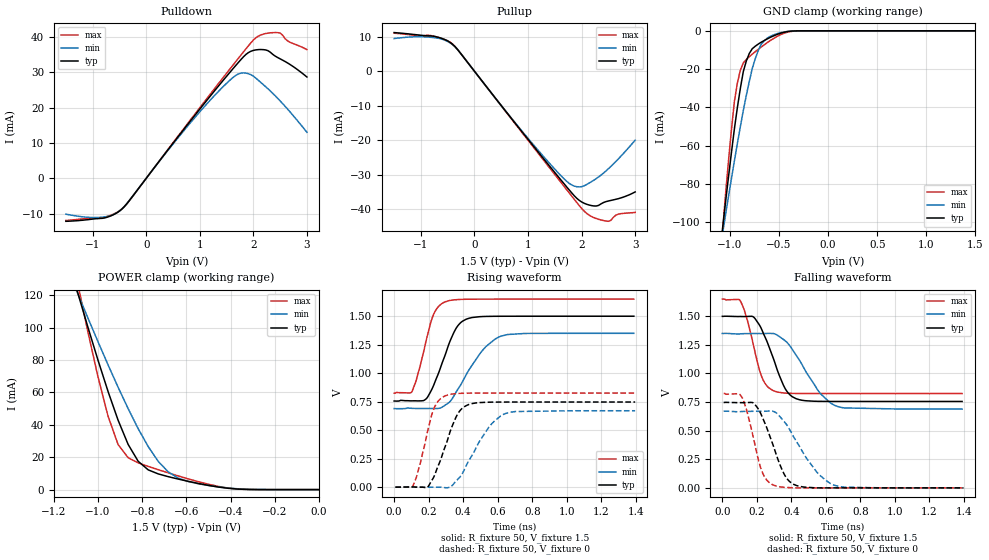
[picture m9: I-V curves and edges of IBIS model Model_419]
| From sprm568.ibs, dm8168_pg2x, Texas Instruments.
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| Model based on original model for BSHTLTCSCDDVGPBFZ
|   Sub model SLOW_8MA_10PER_N_1P5
[model]   Model_419
|[Description]  [1.5V-3-STATE-X-SLOW:8MA, IND, 10%]
|   Slow slew rate (SR[1:0] = "01"), 1.00 * RExt = 1.000 * Iout
|   (I[2:0] = "011"), 8mA nominal with Rext = 50R, ,Industrial
|   temperature range (-40C to 125C, 25C nominal),10% power supply
|   tolerance
|[Input Load]
|[Output Drive] SLOW:8MA
|Voltage   1.5V
|Mode   3-STATE
Model_type   3-state
Polarity   Non-Inverting
Enable   Active-Low
Cref =  15.0000pF
Rref =  100.0000M
Vref =  0V
Vmeas =  0.75
C_comp   1.5249p   1.4275p   1.6205p
[Model Spec]
[Temperature Range]   25   125   -40
[Voltage Range]   1.5   1.35   1.65
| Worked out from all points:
|   slope of the pulldown table from 0 to 0.225 V, typ, clamps not added: 50.1 ohm
|   slope of the pullup table from 0 to 0.225 V, typ, clamps not added: 50.1 ohm
|   GND clamp passes 1 mA (typ) near -0.47 V on its own axis
|   POWER clamp passes 1 mA (typ) near -0.42 V on its own axis
|   rising waveform, R_fixture 50, V_fixture 1.5: 20-80 % time 112ps typ, 168ps min, 83.6ps max; typ from 0.756 V to 1.5 V
|   rising waveform, R_fixture 50, V_fixture 0: 20-80 % time 108ps typ, 154ps min, 80.5ps max; typ from 0 V to 0.747 V
|   falling waveform, R_fixture 50, V_fixture 1.5: 20-80 % time 114ps typ, 168ps min, 82.8ps max; typ from 1.5 V to 0.755 V
|   falling waveform, R_fixture 50, V_fixture 0: 20-80 % time 111ps typ, 170ps min, 80.4ps max; typ from 0.746 V to 0 V
[POWER_clamp]
-1.5V     321.6mA    260.6mA    415.8mA
-1.091V   121.1mA    120.8mA    126.6mA
-1.076V   114.1mA    115.8mA    116.8mA
-1V       79.88mA    91.3mA     69.56mA
-954.5mV  60.58mA    77.05mA    45.34mA
-909.1mV  42.84mA    63.2mA     27.8mA
-818.2mV  17.47mA    37.6mA     16.51mA
-772.7mV  12.19mA    26.53mA    14.33mA
-681.8mV  7.985mA    10.89mA    10.33mA
-590.9mV  5.092mA    4.952mA    6.596mA
-363.6mV  298.9uA    465.6uA    298.1uA
0V        1.518nA    23.05nA    396.5pA
[Pulldown]
-1.5V     -12.15mA   -10.14mA   -11.93mA
-772.7mV  -11.18mA   -10.9mA    -10.98mA
-590.9mV  -10.12mA   -10.11mA   -9.968mA
-409.1mV  -8.017mA   -7.951mA   -8.019mA
954.5mV   18.69mA    17.99mA    19.06mA
1.455V    28.01mA    26.18mA    28.82mA
1.727V    32.86mA    29.54mA    34.05mA
2V        36.15mA    28.87mA    39.08mA
2.318V    35.62mA    24.67mA    41.12mA
2.5V      33.77mA    21.88mA    41.05mA
2.636V    32.63mA    19.61mA    38.86mA
3V        28.64mA    13.01mA    36.37mA
[Pullup]
-1.5V     11.21mA    9.48mA     11.04mA
-772.7mV  10.17mA    9.762mA    10.21mA
-409.1mV  7.827mA    7.7mA      7.892mA
1.227V    -24.14mA   -23.61mA   -24.51mA
1.682V    -32.78mA   -31.32mA   -33.54mA
1.864V    -36.09mA   -33.28mA   -37.13mA
2V        -37.87mA   -33.46mA   -39.75mA
2.182V    -38.93mA   -32.03mA   -42.07mA
2.409V    -38.05mA   -29.51mA   -43.28mA
2.545V    -37.45mA   -27.6mA    -43.23mA
2.682V    -36.95mA   -25.48mA   -41.44mA
3V        -34.98mA   -19.98mA   -40.92mA
[GND_clamp]
-1.5V     -310mA     -250.5mA   -402.4mA
-1.076V   -103.5mA   -106.1mA   -105.2mA
-1.045V   -89.74mA   -96.32mA   -85.93mA
-954.5mV  -51.19mA   -67.85mA   -36.85mA
-924.2mV  -40.06mA   -58.84mA   -27.27mA
-863.6mV  -21.23mA   -41.55mA   -16.73mA
-833.3mV  -15.79mA   -33.74mA   -15.03mA
-772.7mV  -9.342mA   -19.74mA   -12.19mA
-712.1mV  -6.927mA   -10.35mA   -9.702mA
-621.2mV  -4.26mA    -3.894mA   -6.224mA
-409.1mV  -336.9uA   -288.9uA   -618.6uA
1.5V      1.518nA    2.298uA    269.6pA
[Ramp]
dV/dt_f   0.595976/0.16740119n   0.529656/0.25167654n   0.660776/0.12646973n
dV/dt_r 0.60146504/0.15903286n 0.54130904/0.23504658n 0.66263744/0.1220042n
R_load = 50
[Rising Waveform]
R_fixture = 50
V_fixture = 1.5
V_fixture_min = 1.35
V_fixture_max = 1.65
0s        755.8mV    689.4mV    824.8mV
103.1ps   757.4mV    691.6mV    839mV
174.7ps   762.7mV    689.7mV    1.211V
222.4ps   871.1mV    690.6mV    1.492V
299.2ps   1.174V     723.4mV    1.628V
350.8ps   1.371V     812.4mV    1.644V
396.6ps   1.457V     927.5mV    1.648V
521.8ps   1.498V     1.217V     1.65V
617.2ps   1.5V       1.324V     1.65V
1.389ns   1.5V       1.35V      1.65V
[Rising Waveform]
R_fixture = 50
V_fixture = 0
V_fixture_min = 0
V_fixture_max = 0
7.44ps    0V         0V         0V
108.8ps   2.25mV     2.527mV    8.912mV
190.1ps   -2.928mV   0V         464.7mV
225.2ps   76.13mV    0V         668mV
297ps     361.2mV    -4.723mV   802.3mV
361.2ps   622.4mV    57.36mV    821.1mV
405.4ps   704.8mV    148.8mV    824.2mV
548.2ps   745.6mV    524.5mV    825.9mV
645.9ps   746.9mV    646.5mV    826mV
1.396ns   747.2mV    670.5mV    826mV
[Falling Waveform]
R_fixture = 50
V_fixture = 1.5
V_fixture_min = 1.35
V_fixture_max = 1.65
0s        1.499V     1.349V     1.649V
104.7ps   1.498V     1.346V     1.632V
178ps     1.496V     1.349V     1.261V
225.5ps   1.393V     1.348V     981.5mV
294.1ps   1.137V     1.349V     849.7mV
353.3ps   898.8mV    1.298V     829.6mV
405.9ps   795.9mV    1.208V     825.6mV
558.8ps   756.1mV    841.8mV    824.3mV
654.4ps   755.3mV    718.5mV    824.2mV
1.389ns   755.1mV    688.5mV    824.1mV
[Falling Waveform]
R_fixture = 50
V_fixture = 0
V_fixture_min = 0
V_fixture_max = 0
7.44ps    746.3mV    669.6mV    825.4mV
115.9ps   744.4mV    667.7mV    785.8mV
179.6ps   741.4mV    669.2mV    438.6mV
226.1ps   636.7mV    668.8mV    157.6mV
290.5ps   388.1mV    669.8mV    27.86mV
344.8ps   162.4mV    602.8mV    6.921mV
393.3ps   50.43mV    499.8mV    2.104mV
544.6ps   0V         142.4mV    0V
641.1ps   0V         27.55mV    0V
1.396ns   0V         0V         0V
